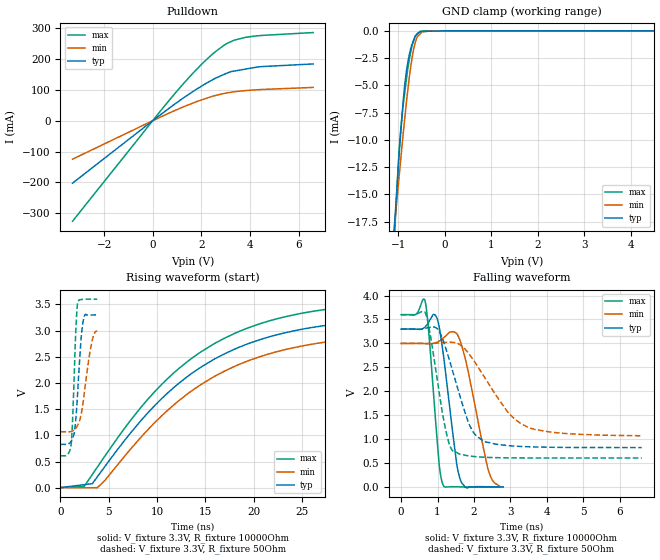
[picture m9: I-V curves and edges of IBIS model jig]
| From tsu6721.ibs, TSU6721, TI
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|   jig Model
[Model]   jig
Model_type   Open_drain
Polarity   Inverting
Vmeas = 1.65
Vref = 3.3
Cref = 2pF
Rref = 10000
|   typ   min   max
C_comp   1.469e-12   1.460e-12   1.761e-12
[Voltage Range]   3.3   3   3.6
|Ambient Temperature   25   85   -40
|Junction Temperature
[Temperature Range]   27   125   -40
[Pullup Reference]   3.3   3   3.6
[Pulldown Reference]   0   0   0
[Power Clamp Reference]   3.3   3   3.6
[GND Clamp Reference]   0   0   0
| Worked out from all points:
|   slope of the pulldown table from 0 to 0.495 V, typ, clamps not added: 16.6 ohm
|   GND clamp passes 1 mA (typ) near -0.68 V on its own axis
|   falling waveform, V_fixture 3.3V, R_fixture 10000Ohm: 20-80 % time 314ps typ, 475ps min, 220ps max; typ from 3.3 V to 0.008 V
|   rising waveform, V_fixture 3.3V, R_fixture 10000Ohm: 20-80 % time 12.3ns typ, 12.4ns min, 12.2ns max; typ from 0.005 V to 3.3 V
|   falling waveform, V_fixture 3.3V, R_fixture 50Ohm: 20-80 % time 599ps typ, 1.05ns min, 382ps max; typ from 3.3 V to 0.829 V
|   rising waveform, V_fixture 3.3V, R_fixture 50Ohm: 20-80 % time 525ps typ, 869ps min, 358ps max; typ from 0.83 V to 3.3 V
[Pulldown]
|   Voltage   I(typ)   I(min)   I(max)
-3.3V     -202.6mA   -124.8mA   -326.2mA
172.8mV   10.55mA    6.376mA    17.16mA
939.6mV   55.69mA    33.9mA     90.61mA
1.706V    97.16mA    58.76mA    158.3mA
2.538V    136mA      80.85mA    221.4mA
3.089V    155.4mA    90.6mA     251.9mA
3.355V    161mA      93.76mA    261.2mA
3.812V    167.3mA    97.58mA    270.2mA
4.5V      175.5mA    101.2mA    276.6mA
6.6V      184.1mA    107.9mA    285.8mA
[GND Clamp]
|   Voltage   I(typ)   I(min)   I(max)
-3.3V     -190.1mA   -129.9mA   -289.9mA
-1.102V   -19.23mA   -18.86mA   -21.26mA
-1.066V   -16.8mA    -17.13mA   -17.5mA
-986.4mV  -11.53mA   -13.55mA   -11.2mA
-946.8mV  -9.312mA   -11.76mA   -8.992mA
-897.6mV  -6.559mA   -9.547mA   -6.883mA
-828.3mV  -3.801mA   -6.687mA   -4.556mA
-745.8mV  -1.854mA   -3.713mA   -2.238mA
-678mV    -963.4uA   -1.843mA   -971.7uA
-600mV    -301uA     -627.7uA   -323.1uA
-532.8mV  -103uA     -290.7uA   -52.67uA
6.6V      0A         0A         0A
[POWER Clamp]
|   Voltage   I(typ)   I(min)   I(max)
-3.3V     0A         0A         0A
0V        0A         0A         0A
6.6V      0A         0A         0A
[Ramp]
R_load = 10000
|   typ   min   max
dV/dt_r   1.97677/1.23097e-08   1.79521/1.24571e-08   2.15783/1.22152e-08
dV/dt_f   1.97678/3.14059e-10   1.79523/4.74438e-10   2.15784/2.19994e-10
[Falling Waveform]
V_fixture = 3.3V
V_fixture_min = 3V
V_fixture_max = 3.6V
R_fixture = 10000Ohm
|   Time   V(typ)   V(min)   V(max)
0s        3.3V       3V         3.6V
650ps     3.337V     2.998V     3.913V
750ps     3.434V     2.996V     3.326V
950ps     3.579V     3.016V     1.362V
1.05ns    3.328V     3.051V     443mV
1.175ns   2.682V     3.124V     15.14mV
1.525ns   492.6mV    3.211V     10.89mV
1.65ns    112.8mV    2.991V     8.897mV
2.4ns     11.36mV    338.5mV    4.685mV
2.8ns     8.48mV     7.275mV    4.009mV
[Rising Waveform]
V_fixture = 3.3V
V_fixture_min = 3V
V_fixture_max = 3.6V
R_fixture = 10000Ohm
|   Time   V(typ)   V(min)   V(max)
0s        5.366mV    7.912mV    3.602mV
2.45ns    61.08mV    1.58mV     26.4mV
3.3ns     80.41mV    2.987mV    255.6mV
3.825ns   212.9mV    3.855mV    397.8mV
8.25ns    1.266V     950mV      1.518V
11.83ns   1.93V      1.598V     2.209V
15.9ns    2.454V     2.123V     2.75V
20.58ns   2.824V     2.499V     3.128V
32.63ns   3.197V     2.884V     3.501V
57.65ns   3.296V     2.994V     3.596V
[Falling Waveform]
V_fixture = 3.3V
V_fixture_min = 3V
V_fixture_max = 3.6V
R_fixture = 50Ohm
|   Time   V(typ)   V(min)   V(max)
0s        3.3V       3V         3.6V
675ps     3.317V     2.999V     3.623V
1.05ns    3.247V     3.011V     1.96V
1.3ns     2.72V      3.025V     959.4mV
1.45ns    2.331V     3.02V      737.7mV
1.875ns   1.301V     2.77V      654.1mV
2.3ns     952.1mV    2.283V     626.3mV
2.95ns    868.7mV    1.55V      614.3mV
3.525ns   844.3mV    1.239V     611.7mV
6.6ns     828.9mV    1.075V     611.5mV
[Rising Waveform]
V_fixture = 3.3V
V_fixture_min = 3V
V_fixture_max = 3.6V
R_fixture = 50Ohm
|   Time   V(typ)   V(min)   V(max)
0s        829.6mV    1.071V     611.5mV
1.125ns   893.3mV    1.076V     859.3mV
1.25ns    936.6mV    1.085V     1.268V
1.475ns   1.108V     1.116V     2.428V
1.675ns   1.51V      1.161V     3.305V
1.8ns     1.878V     1.2V       3.543V
2.15ns    2.877V     1.409V     3.593V
2.45ns    3.261V     1.785V     3.601V
3.275ns   3.299V     2.803V     3.6V
3.8ns     3.301V     2.989V     3.6V
